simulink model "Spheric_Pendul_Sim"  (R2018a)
settings: Solver=ode8  StartTime=0.0  StopTime=80  FixedStep=Ts  MaxStep=0.0001  RelTol=1e-6  EnableMultiTasking=on
InitFcn:
  | init
StopFcn:
  | pl2
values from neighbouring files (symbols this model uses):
  Ax = 54.8    [init.m]
  d2r = pi/180    (= 0.0174532925199)    [init.m]
  Ixx = 3561    [init.m]
  Iyy = 20921    [init.m]
  Izz = 20763    [init.m]
  Mlh2 = 41.12    [init.m]
  Mlox = 119.3    [init.m]
  phi0 = 45*d2r    (= 0.785398163397)    [init.m]
  phid0 = 200.0*d2r    (= 3.49065850399)    [init.m]
  Rsl = 2.5    [init.m]
  thet0 = 18.0*d2r    (= 0.314159265359)    [init.m]
  Thr = 3.0    (= 3)    [init.m]
  x1_ini = [-1,0, -2,0, 2,0]*d2r    [init.m]
  x3_ini = [x1_ini,x3_ini]    [init.m]
  Xcg = 91.75    [init.m]
  Ys0 = R0*cos(phi0)    [init.m]
  Zeta = 0.002    [init.m]
  Zs0 = -R0*sin(phi0)    [init.m]
undefined symbols (not defined in the file or in its folder): Av2, Bv2, Cv2, Dv2, Kmix, Kq

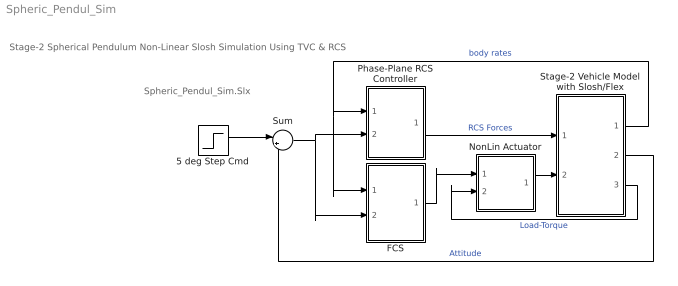
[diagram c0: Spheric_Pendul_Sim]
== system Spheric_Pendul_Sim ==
  note: Stage-2 Spherical Pendulum Non-Linear Slosh Simulation Using TVC & RCS
  note: Spheric_Pendul_Sim.Slx
  5 deg Step Cmd : Step  Time=0  Before=[0,0,0]  After=[1, 1, -1]*d2r*5  SampleTime=0
  FCS : Subsystem
  NonLin Actuator : Subsystem
  Phase-Plane RCS Controller : Subsystem
  Stage-2 Vehicle Model with Slosh/Flex : Subsystem
  Sum : Sum  Inputs=|+-
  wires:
  Stage-2 Vehicle Model with Slosh/Flex/1(Wb) -> Phase-Plane RCS Controller/1(rate), FCS/1(rate)  "body rates"
  Sum/1 -> Phase-Plane RCS Controller/2(atter), FCS/2(atter)
  Stage-2 Vehicle Model with Slosh/Flex/2(atti) -> Sum/2  "Attitude"
  FCS/1(DQ,DR) -> NonLin Actuator/1(dc)
  5 deg Step Cmd/1 -> Sum/1
  Stage-2 Vehicle Model with Slosh/Flex/3(TL) -> NonLin Actuator/2(TL)  "Load-Torque"
  Phase-Plane RCS Controller/1(f(i)) -> Stage-2 Vehicle Model with Slosh/Flex/1(Frcs)  "RCS Forces"
  NonLin Actuator/1(del) -> Stage-2 Vehicle Model with Slosh/Flex/2(dy,dz)

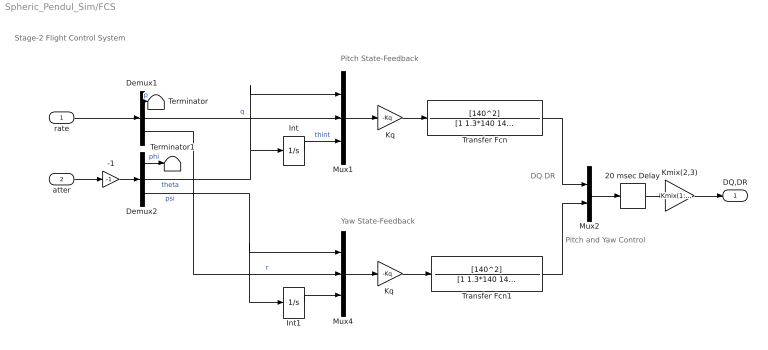
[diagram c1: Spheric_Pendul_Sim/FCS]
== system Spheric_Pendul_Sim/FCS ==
  note: DQ DR
  note: Pitch State-Feedback
  note: Yaw State-Feedback
  note: Pitch and Yaw Control
  note: Stage-2 Flight Control System
  rate : Inport
  atter : Inport  Port=2
  -1 : Gain  Gain=-1
  20 msec Delay : TransportDelay  DelayTime="[1  1]*0.020"  InitialOutput=[0 0]  PadeOrder=2
  Demux1 : Demux  Outputs=3
  Demux2 : Demux  Outputs=3
  Int : Integrator
  Int1 : Integrator
  Kmix(2,3) : Gain  Gain=Kmix(1:2,2:3)  Multiplication=Matrix(K*u)
  Kq : Gain  Gain=-Kq  Multiplication=Matrix(K*u)
  "Kq " : Gain  Gain=-Kq  Multiplication=Matrix(K*u)
  Mux1 : Mux  Inputs=3
  Mux2 : Mux  Inputs=2
  Mux4 : Mux  Inputs=3
  Terminator : Terminator
  Terminator1 : Terminator
  Transfer Fcn : TransferFcn  Numerator=[140^2]  Denominator=[1 1.3*140 140^2]
  Transfer Fcn1 : TransferFcn  Numerator=[140^2]  Denominator=[1 1.3*140 140^2]
  DQ,DR : Outport
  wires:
  Mux2/1 -> 20 msec Delay/1
  rate/1 -> Demux1/1
  Kq/1 -> Transfer Fcn/1
  Demux2/2 -> Mux1/1, Int/1  "theta"
  Demux1/2 -> Mux1/2  "q"
  Int/1 -> Mux1/3  "thint"
  Int1/1 -> Mux4/3
  Demux1/3 -> Mux4/2  "r"
  Demux2/3 -> Int1/1, Mux4/1  "psi"
  atter/1 -> -1/1
  Mux1/1 -> Kq/1
  Transfer Fcn/1 -> Mux2/1
  Transfer Fcn1/1 -> Mux2/2
  Mux4/1 -> "Kq "/1
  "Kq "/1 -> Transfer Fcn1/1
  Demux1/1 -> Terminator/1  "p"
  Demux2/1 -> Terminator1/1  "phi"
  20 msec Delay/1 -> Kmix(2,3)/1
  -1/1 -> Demux2/1
  Kmix(2,3)/1 -> DQ,DR/1

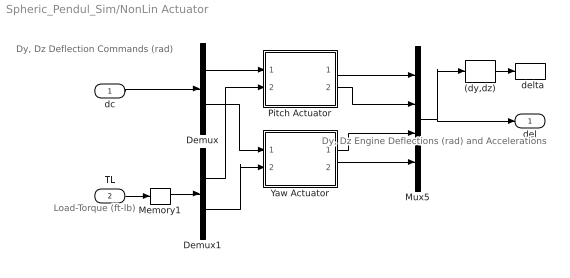
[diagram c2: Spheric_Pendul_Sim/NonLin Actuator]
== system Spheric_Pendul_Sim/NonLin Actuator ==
  note: Load-Torque (ft-lb)
  note: Dy, Dz Deflection Commands (rad)
  note: Dy, Dz Engine Deflections (rad) and Accelerations
  dc : Inport
  TL : Inport  Port=2
  "  delta" : ToWorkspace  VariableName=delta  SampleTime=-1
  (dy,dz) : Selector  InputPortWidth=4  IndexOptions=Index vector (dialog)  Indices=[1,3]  OutputSizes=1
  Demux : Demux  Outputs=2
  Demux1 : Demux  Outputs=2
  Memory1 : Memory
  Mux5 : Mux
  Pitch Actuator : Subsystem
  Yaw Actuator : Subsystem
  del : Outport
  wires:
  TL/1 -> Memory1/1
  dc/1 -> Demux/1
  Yaw Actuator/2(ddot) -> Mux5/4
  Demux/1 -> Pitch Actuator/1(delc)
  Pitch Actuator/2(ddot) -> Mux5/2
  Demux/2 -> Yaw Actuator/1(delc)
  Demux1/2 -> Yaw Actuator/2(TL)
  Mux5/1 -> del/1, (dy,dz)/1
  Demux1/1 -> Pitch Actuator/2(TL)
  (dy,dz)/1 -> "  delta"/1
  Memory1/1 -> Demux1/1
  Yaw Actuator/1(del) -> Mux5/3
  Pitch Actuator/1(del) -> Mux5/1

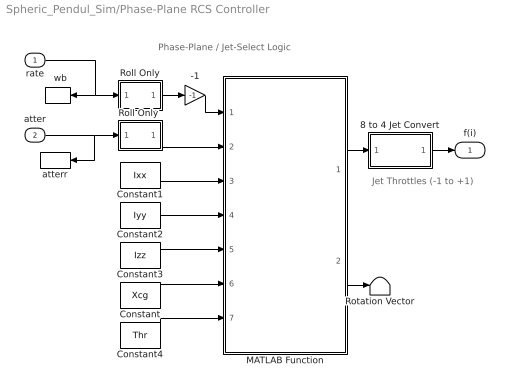
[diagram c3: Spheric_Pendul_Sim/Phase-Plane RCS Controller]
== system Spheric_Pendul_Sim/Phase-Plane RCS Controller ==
  note: Phase-Plane / Jet-Select Logic
  note: Jet Throttles (-1 to +1)
  rate : Inport
  atter : Inport  Port=2
  "  wb" : ToWorkspace  VariableName=wb  SampleTime=-1
  -1 : Gain  Gain=-1
  8 to 4 Jet Convert : Subsystem
  Constant : Constant  Value=Xcg
  Constant1 : Constant  Value=Ixx
  Constant2 : Constant  Value=Iyy
  Constant3 : Constant  Value=Izz
  Constant4 : Constant  Value=Thr
  MATLAB Function : MATLAB Function  TreatAsAtomicUnit=on
  Roll Only : Subsystem
  "Roll Only " : Subsystem
  Rotation Vector : Terminator
  atterr : ToWorkspace  VariableName=atter  SampleTime=-1
  f(i) : Outport
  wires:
  MATLAB Function/2(eu) -> Rotation Vector/1
  Constant4/1 -> MATLAB Function/7(Thr)
  Constant3/1 -> MATLAB Function/5(J33)
  8 to 4 Jet Convert/1(f(4)) -> f(i)/1
  MATLAB Function/1(fp) -> 8 to 4 Jet Convert/1(f(8))
  Constant2/1 -> MATLAB Function/4(J22)
  Constant1/1 -> MATLAB Function/3(J11)
  rate/1 -> "  wb"/1, Roll Only/1(w)
  Constant/1 -> MATLAB Function/6(Xcg)
  -1/1 -> MATLAB Function/1(Rater)
  Roll Only/1(p) -> -1/1
  "Roll Only "/1(p) -> MATLAB Function/2(Atter)
  atter/1 -> "Roll Only "/1(w), atterr/1

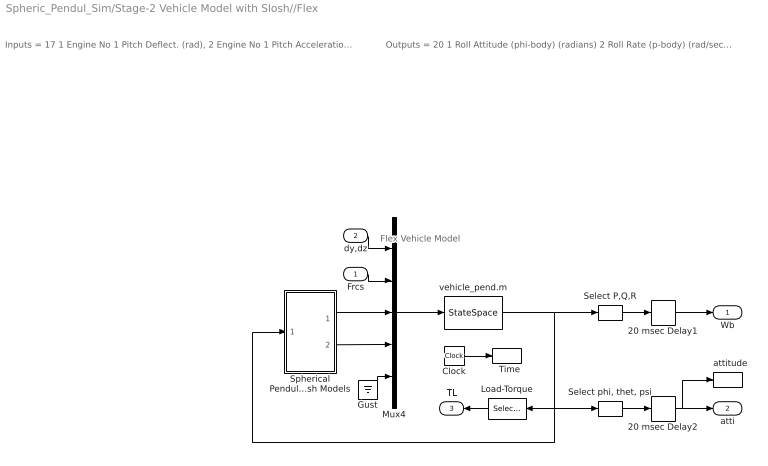
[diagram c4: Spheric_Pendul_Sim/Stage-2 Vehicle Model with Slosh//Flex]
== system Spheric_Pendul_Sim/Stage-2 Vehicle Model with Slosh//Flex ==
  note: Flex Vehicle Model
  note: Inputs = 17 1 Engine No 1 Pitch Deflect. (rad), 2 Engine No 1 Pitch Acceleration (rad/sec^2) 3 Engine No 1 Yaw Deflect. (rad), 4 Engine No 1 Yaw Acceleration (rad/sec^2) 5 RCS 1 Throttle Input dTh/Th 6 RCS 2 Throttle Input dTh/Th 7 RCS 3 Throttle Input dTh/Th 8 RCS 4 Throttle Input dTh/Th 9 LOX Force along Y-axis 10 LOX Force along Z-axis 11 LH2 Force along Y-axis 12 LH2 Force along Z-axis 13 Ext LOX Pitch Torque Inp 1 (ft-lb) 14 Ext LOX Yaw Torque Input 2 (ft-lb) 15 Ext LH2 Pitch Torque Inp 3 (ft-lb) 16 Ext LH2 Yaw Torque Input 4 (ft-lb) 17 Wind Gust Velocity (ft/sec)
  note: Outputs = 20 1 Roll Attitude (phi-body) (radians) 2 Roll Rate (p-body) (rad/sec) 3 Pitch Attitude (thet-bdy) (radians) 4 Pitch Rate (q-body) (rad/sec) 5 Yaw Attitude (psi-body) (radians) 6 Yaw Rate (r-body) (rad/sec) 7 Angle of attack, alfa, (radians) 8 Angle of sideslip, beta, (radian) 9 Change in Altitude, delta-h, (feet) 10 Forward Acceleration (V-dot) (ft/sec) 11 Cross Range Velocity (Vcr) (ft/sec) 12 Rate-Gyro # 1, Roll Rate (Body) (rad/sec) 13 Rate-Gyro # 2, Pitch Rate (Body) (rad/sec) 14 Rate-Gyro # 3, Yaw Rate (Body) (rad/sec) 15 Accelerat # 1, at LOX (along Y), (ft/sec^2) 16 Accelerat # 2, at LOX (along Z), (ft/sec^2) 17 Accelerat # 3, at LH2 (along Y), (ft/sec^2) 18 Accelerat # 4, at LH2 (along Z), (ft/sec^2) 19 Ptch Engine Load-Torque Tly (ft-lb) 20 Yaw Engine Load-Torque Tlz (ft-lb)
  Frcs : Inport
  dy,dz : Inport  Port=2
  "  Time" : ToWorkspace  VariableName=tim  SampleTime=-1
  "  attitude" : ToWorkspace  VariableName=atti  SampleTime=-1
  20 msec Delay1 : TransportDelay  DelayTime=[1 1 1]*0.02  InitialOutput=[0 0 0]  PadeOrder=2
  20 msec Delay2 : TransportDelay  DelayTime=[1 1 1]*0.02  InitialOutput=x1_ini([1,3,5])  PadeOrder=2
  Clock : Clock
  Gust : Ground
  Load-Torque : Selector  InputPortWidth=20  IndexOptions=Index vector (dialog)  Indices=[19, 20]  OutputSizes=1
  Mux4 : Mux  Inputs=[4,4,4,4,1]
  Select P,Q,R : Selector  InputPortWidth=20  IndexOptions=Index vector (dialog)  Indices=[12,13,14]  OutputSizes=1
  "Select phi, thet, psi" : Selector  InputPortWidth=20  IndexOptions=Index vector (dialog)  Indices=[1,3,5]  OutputSizes=1
  Spherical Pendulum Slosh Models : Subsystem
  vehicle_pend.m : StateSpace  A=Av2  B=Bv2  C=Cv2  D=Dv2  InitialCondition=x3_ini
  Wb : Outport
  atti : Outport  Port=2
  TL : Outport  Port=3
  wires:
  Gust/1 -> Mux4/5
  Frcs/1 -> Mux4/2
  dy,dz/1 -> Mux4/1
  Load-Torque/1 -> TL/1
  Clock/1 -> "  Time"/1
  20 msec Delay2/1 -> "  attitude"/1, atti/1
  20 msec Delay1/1 -> Wb/1
  vehicle_pend.m/1 -> Select P,Q,R/1, "Select phi, thet, psi"/1, Spherical Pendulum Slosh Models/1(Ayz), Load-Torque/1
  Spherical Pendulum Slosh Models/1(Fyz) -> Mux4/3
  Spherical Pendulum Slosh Models/2(Myz) -> Mux4/4
  Select P,Q,R/1 -> 20 msec Delay1/1
  "Select phi, thet, psi"/1 -> 20 msec Delay2/1
  Mux4/1 -> vehicle_pend.m/1

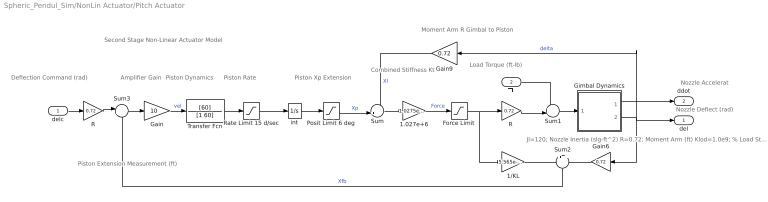
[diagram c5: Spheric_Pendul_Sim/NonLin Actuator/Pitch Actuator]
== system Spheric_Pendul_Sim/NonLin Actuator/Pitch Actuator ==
  note: Jl=120; Nozzle Inertia (slg-ft^2) R=0.72; Moment Arm (ft) Klod=1.0e9; % Load Stiffness Kact=2.4e6; % Piston Stiffness Kbck=1.13e6; % Backup Structure Stiffn Kti=(1/Klod)+(1/Kact)+(1/Kbck); Kt=1/Kti; % Combined Structural Stiffness Ka=8; % Amplifier Gain
  note: Load Torque (ft-lb)
  note: Deflection Command (rad)
  note: Piston Xp Extension
  note: Combined Stiffness Kt
  note: Piston Dynamics
  note: Nozzle Accelerat
  note: Nozzle Deflect (rad)
  note: Amplifier Gain
  note: Piston Rate
  note: Second Stage Non-Linear Actuator Model
  note: Moment Arm R Gimbal to Piston
  note: Piston Extension Measurement (ft)
  delc : Inport
  TL : Inport  Port=2
  1.027e+6 : Gain  Gain=1.0275e+6
  1/KL : Gain  Gain=5.565e-07
  Force Limit : Saturate  UpperLimit=4000  LowerLimit=-4000
  Gain : Gain  Gain=10
  Gain6 : Gain  Gain=0.72
  Gain9 : Gain  Gain=0.72
  Gimbal Dynamics : Subsystem
  Posit Limit 6 deg : Saturate  UpperLimit=0.075  LowerLimit=-0.075
  R : Gain  Gain=0.72
  "R " : Gain  Gain=0.72
  Rate Limit 15 d/sec : Saturate  UpperLimit=0.125  LowerLimit=-0.125
  Sum : Sum  Inputs=-+|
  Sum1 : Sum  Inputs=++|
  Sum2 : Sum  Inputs=+|+
  Sum3 : Sum  Inputs=|+-
  Transfer Fcn : TransferFcn  Numerator=[60]  Denominator=[1 60]
  int : Integrator
  del : Outport
  ddot : Outport  Port=2
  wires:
  Transfer Fcn/1 -> Rate Limit 15 d/sec/1
  Sum1/1 -> Gimbal Dynamics/1(Tin)
  Gimbal Dynamics/1(Axel) -> ddot/1
  Posit Limit 6 deg/1 -> Sum/2  "Xp"
  1/KL/1 -> Sum2/1
  Gain9/1 -> Sum/1  "Xl"
  1.027e+6/1 -> Force Limit/1  "Force"
  Gain6/1 -> Sum2/2
  Rate Limit 15 d/sec/1 -> int/1
  Gain/1 -> Transfer Fcn/1  "vel"
  Sum3/1 -> Gain/1
  Sum/1 -> 1.027e+6/1
  int/1 -> Posit Limit 6 deg/1
  TL/1 -> Sum1/1
  R/1 -> Sum3/1
  delc/1 -> R/1
  Force Limit/1 -> "R "/1, 1/KL/1
  "R "/1 -> Sum1/2
  Gimbal Dynamics/2(" delta") -> Gain9/1, del/1, Gain6/1  "delta"
  Sum2/1 -> Sum3/2  "Xfb"

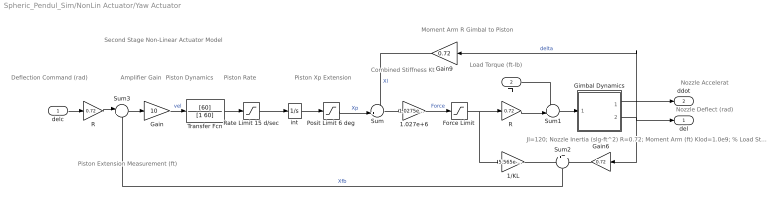
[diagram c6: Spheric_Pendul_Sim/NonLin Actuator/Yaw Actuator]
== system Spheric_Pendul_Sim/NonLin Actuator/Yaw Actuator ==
  note: Jl=120; Nozzle Inertia (slg-ft^2) R=0.72; Moment Arm (ft) Klod=1.0e9; % Load Stiffness Kact=2.4e6; % Piston Stiffness Kbck=1.13e6; % Backup Structure Stiffn Kti=(1/Klod)+(1/Kact)+(1/Kbck); Kt=1/Kti; % Combined Structural Stiffness Ka=8; % Amplifier Gain
  note: Load Torque (ft-lb)
  note: Deflection Command (rad)
  note: Piston Xp Extension
  note: Combined Stiffness Kt
  note: Piston Dynamics
  note: Nozzle Accelerat
  note: Nozzle Deflect (rad)
  note: Amplifier Gain
  note: Piston Rate
  note: Second Stage Non-Linear Actuator Model
  note: Moment Arm R Gimbal to Piston
  note: Piston Extension Measurement (ft)
  delc : Inport
  TL : Inport  Port=2
  1.027e+6 : Gain  Gain=1.0275e+6
  1/KL : Gain  Gain=5.565e-07
  Force Limit : Saturate  UpperLimit=4000  LowerLimit=-4000
  Gain : Gain  Gain=10
  Gain6 : Gain  Gain=0.72
  Gain9 : Gain  Gain=0.72
  Gimbal Dynamics : Subsystem
  Posit Limit 6 deg : Saturate  UpperLimit=0.075  LowerLimit=-0.075
  R : Gain  Gain=0.72
  "R " : Gain  Gain=0.72
  Rate Limit 15 d/sec : Saturate  UpperLimit=0.125  LowerLimit=-0.125
  Sum : Sum  Inputs=-+|
  Sum1 : Sum  Inputs=++|
  Sum2 : Sum  Inputs=+|+
  Sum3 : Sum  Inputs=|+-
  Transfer Fcn : TransferFcn  Numerator=[60]  Denominator=[1 60]
  int : Integrator
  del : Outport
  ddot : Outport  Port=2
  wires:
  Transfer Fcn/1 -> Rate Limit 15 d/sec/1
  Sum1/1 -> Gimbal Dynamics/1(Tin)
  Gimbal Dynamics/1(Axel) -> ddot/1
  Posit Limit 6 deg/1 -> Sum/2  "Xp"
  1/KL/1 -> Sum2/1
  Gain9/1 -> Sum/1  "Xl"
  1.027e+6/1 -> Force Limit/1  "Force"
  Gain6/1 -> Sum2/2
  Rate Limit 15 d/sec/1 -> int/1
  Gain/1 -> Transfer Fcn/1  "vel"
  Sum3/1 -> Gain/1
  Sum/1 -> 1.027e+6/1
  int/1 -> Posit Limit 6 deg/1
  TL/1 -> Sum1/1
  R/1 -> Sum3/1
  delc/1 -> R/1
  Force Limit/1 -> "R "/1, 1/KL/1
  "R "/1 -> Sum1/2
  Gimbal Dynamics/2(" delta") -> Gain9/1, del/1, Gain6/1  "delta"
  Sum2/1 -> Sum3/2  "Xfb"

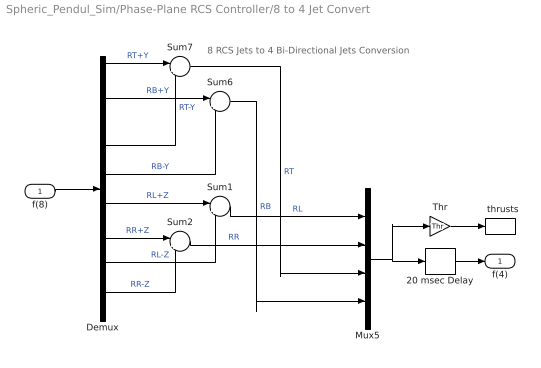
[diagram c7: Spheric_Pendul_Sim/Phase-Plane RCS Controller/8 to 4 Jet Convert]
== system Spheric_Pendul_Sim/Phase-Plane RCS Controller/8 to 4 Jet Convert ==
  note: 8 RCS Jets to 4 Bi-Directional Jets Conversion
  f(8) : Inport
  "  thrusts" : ToWorkspace  VariableName=Jets  SampleTime=-1
  20 msec Delay : TransportDelay  DelayTime="[1  1  1  1]*0.020"  InitialOutput="[0  0  0  0]"  PadeOrder=2
  Demux : Demux  Outputs=8
  Mux5 : Mux
  Sum{1..2,6..7} (4 alike) : Sum  Inputs=|+-
  Thr : Gain  Gain=Thr
  f(4) : Outport
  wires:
  Thr/1 -> "  thrusts"/1
  20 msec Delay/1 -> f(4)/1
  Sum2/1 -> Mux5/2  "RR"
  Sum1/1 -> Mux5/1  "RL"
  Demux/4 -> Sum6/2  "RB-Y"
  Demux/2 -> Sum6/1  "RB+Y"
  Demux/3 -> Sum7/2  "RT-Y"
  Sum7/1 -> Mux5/3  "RT"
  Demux/8 -> Sum2/2  "RR-Z"
  Demux/5 -> Sum1/1  "RL+Z"
  Sum6/1 -> Mux5/4  "RB"
  Demux/1 -> Sum7/1  "RT+Y"
  Demux/6 -> Sum2/1  "RR+Z"
  Demux/7 -> Sum1/2  "RL-Z"
  Mux5/1 -> Thr/1, 20 msec Delay/1
  f(8)/1 -> Demux/1

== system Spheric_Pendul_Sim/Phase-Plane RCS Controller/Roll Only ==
  w : Inport
  Ground : Ground
  Mux : Mux  Inputs=3
  Selector : Selector  InputPortWidth=3  IndexOptions=Index vector (dialog)  Indices=[1]  OutputSizes=1
  p : Outport
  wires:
  Ground/1 -> Mux/2, Mux/3
  Selector/1 -> Mux/1
  Mux/1 -> p/1
  w/1 -> Selector/1

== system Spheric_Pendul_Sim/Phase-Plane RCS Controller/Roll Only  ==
  w : Inport
  Ground : Ground
  Mux : Mux  Inputs=3
  Selector : Selector  InputPortWidth=3  IndexOptions=Index vector (dialog)  Indices=[1]  OutputSizes=1
  p : Outport
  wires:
  Ground/1 -> Mux/2, Mux/3
  Selector/1 -> Mux/1
  Mux/1 -> p/1
  w/1 -> Selector/1

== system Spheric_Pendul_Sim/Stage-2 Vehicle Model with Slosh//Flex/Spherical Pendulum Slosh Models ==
  note: Spherical Pendulum Slosh Modes
  Ayz : Inport
  LH2 Slosh : Subsystem
  LOX Slosh : Subsystem
  Mux1 : Mux  Inputs=[2, 2]
  Mux2 : Mux  Inputs=[2, 2]
  Fyz : Outport
  Myz : Outport  Port=2
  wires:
  Mux1/1 -> Fyz/1
  LOX Slosh/1(Fox) -> Mux1/1
  LH2 Slosh/1(Fh2) -> Mux1/2
  LOX Slosh/2(Mox) -> Mux2/1
  LH2 Slosh/2(Mh2) -> Mux2/2
  Mux2/1 -> Myz/1
  Ayz/1 -> LH2 Slosh/1(Ayz), LOX Slosh/1(Ayz)

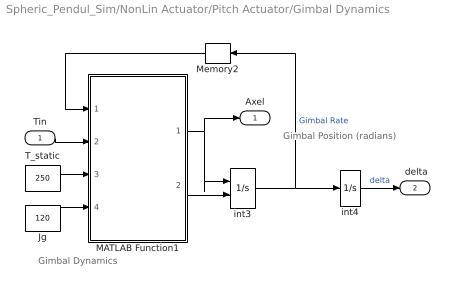
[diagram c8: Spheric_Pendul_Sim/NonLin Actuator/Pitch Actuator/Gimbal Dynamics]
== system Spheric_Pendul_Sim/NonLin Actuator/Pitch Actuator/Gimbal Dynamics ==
  note: Gimbal Dynamics
  note: Gimbal Position (radians)
  Tin : Inport
  Jg : Constant  Value=120
  MATLAB Function1 : MATLAB Function  TreatAsAtomicUnit=on
  Memory2 : Memory
  T_static : Constant  Value=250
  int3 : Integrator  ExternalReset=rising
  int4 : Integrator
  Axel : Outport
  " delta" : Outport  Port=2
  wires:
  Memory2/1 -> MATLAB Function1/1(Rate)
  Jg/1 -> MATLAB Function1/4(Jg)
  MATLAB Function1/1(Axel) -> int3/1, Axel/1
  T_static/1 -> MATLAB Function1/3(Tst)
  Tin/1 -> MATLAB Function1/2(Tin)
  int3/1 -> Memory2/1, int4/1  "Gimbal Rate"
  int4/1 -> " delta"/1  "delta"
  MATLAB Function1/2(Rvel) -> int3/2

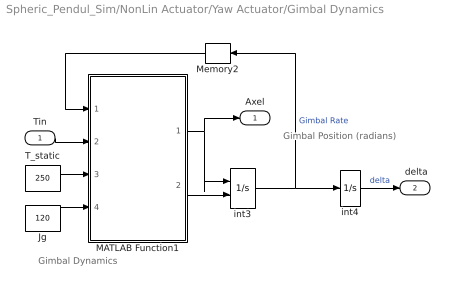
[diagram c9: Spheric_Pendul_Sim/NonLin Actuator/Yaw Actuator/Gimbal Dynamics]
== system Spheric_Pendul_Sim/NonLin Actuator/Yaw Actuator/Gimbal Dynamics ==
  note: Gimbal Dynamics
  note: Gimbal Position (radians)
  Tin : Inport
  Jg : Constant  Value=120
  MATLAB Function1 : MATLAB Function  TreatAsAtomicUnit=on
  Memory2 : Memory
  T_static : Constant  Value=250
  int3 : Integrator  ExternalReset=rising
  int4 : Integrator
  Axel : Outport
  " delta" : Outport  Port=2
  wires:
  Memory2/1 -> MATLAB Function1/1(Rate)
  Jg/1 -> MATLAB Function1/4(Jg)
  MATLAB Function1/1(Axel) -> int3/1, Axel/1
  T_static/1 -> MATLAB Function1/3(Tst)
  Tin/1 -> MATLAB Function1/2(Tin)
  int3/1 -> Memory2/1, int4/1  "Gimbal Rate"
  int4/1 -> " delta"/1  "delta"
  MATLAB Function1/2(Rvel) -> int3/2

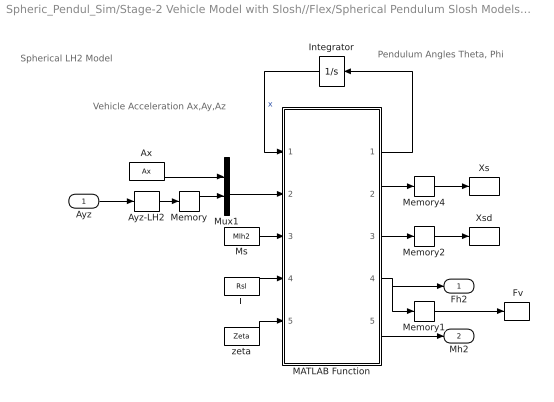
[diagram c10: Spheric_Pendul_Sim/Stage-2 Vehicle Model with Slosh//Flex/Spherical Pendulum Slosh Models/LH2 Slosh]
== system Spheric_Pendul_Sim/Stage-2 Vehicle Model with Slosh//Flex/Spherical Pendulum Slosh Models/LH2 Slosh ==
  note: Spherical LH2 Model
  note: Vehicle Acceleration Ax,Ay,Az
  note: Pendulum Angles Theta, Phi
  Ayz : Inport
  " Fv" : ToWorkspace  VariableName=Fvb  SampleTime=-1
  " Xs " : ToWorkspace  VariableName=Xsb  SampleTime=-1
  " Xsd " : ToWorkspace  VariableName=Xsdb  SampleTime=-1
  Ax : Constant  Value=Ax
  Ayz-LH2 : Selector  InputPortWidth=20  IndexOptions=Index vector (dialog)  Indices=[17,18]  OutputSizes=1
  Integrator : Integrator  InitialCondition=[0,phid0, thet0,phi0]
  L : Constant  Value=Rsl
  MATLAB Function : MATLAB Function  TreatAsAtomicUnit=on
  Memory : Memory
  Memory1 : Memory
  Memory2 : Memory
  Memory4 : Memory  InitialCondition=[Ys0,Zs0]
  Ms : Constant  Value=Mlh2
  Mux1 : Mux  Inputs=[1, 2]
  zeta : Constant  Value=Zeta
  Fh2 : Outport
  Mh2 : Outport  Port=2
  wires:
  MATLAB Function/5(Mv) -> Mh2/1
  MATLAB Function/4(Fv) -> Fh2/1, Memory1/1
  L/1 -> MATLAB Function/4(Rsl)
  zeta/1 -> MATLAB Function/5(zeta)
  Ms/1 -> MATLAB Function/3(Msl)
  Mux1/1 -> MATLAB Function/2(Acc)
  MATLAB Function/1(xdot) -> Integrator/1
  Integrator/1 -> MATLAB Function/1(x)  "x"
  MATLAB Function/2(Xs) -> Memory4/1
  MATLAB Function/3(Xsd) -> Memory2/1
  Memory1/1 -> " Fv"/1
  Memory4/1 -> " Xs "/1
  Memory2/1 -> " Xsd "/1
  Ayz/1 -> Ayz-LH2/1
  Ax/1 -> Mux1/1
  Ayz-LH2/1 -> Memory/1
  Memory/1 -> Mux1/2

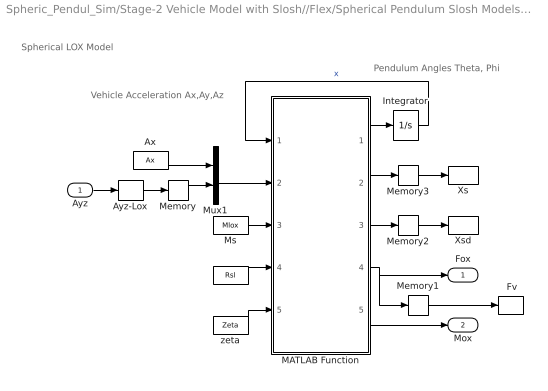
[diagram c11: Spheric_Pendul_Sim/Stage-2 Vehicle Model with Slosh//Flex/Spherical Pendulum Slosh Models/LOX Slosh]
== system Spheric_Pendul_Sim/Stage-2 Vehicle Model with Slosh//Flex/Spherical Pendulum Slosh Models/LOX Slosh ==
  note: Spherical LOX Model
  note: Vehicle Acceleration Ax,Ay,Az
  note: Pendulum Angles Theta, Phi
  Ayz : Inport
  " Fv" : ToWorkspace  VariableName=Fva  SampleTime=-1
  " Xs " : ToWorkspace  VariableName=Xsa  SampleTime=-1
  " Xsd " : ToWorkspace  VariableName=Xsda  SampleTime=-1
  Ax : Constant  Value=Ax
  Ayz-Lox : Selector  InputPortWidth=20  IndexOptions=Index vector (dialog)  Indices=[15,16]  OutputSizes=1
  Integrator : Integrator  InitialCondition=[0,phid0, thet0,phi0]
  L : Constant  Value=Rsl
  MATLAB Function : MATLAB Function  TreatAsAtomicUnit=on
  Memory : Memory
  Memory1 : Memory
  Memory2 : Memory
  Memory3 : Memory  InitialCondition=[Ys0, Zs0]
  Ms : Constant  Value=Mlox
  Mux1 : Mux  Inputs=[1, 2]
  zeta : Constant  Value=Zeta
  Fox : Outport
  Mox : Outport  Port=2
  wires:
  MATLAB Function/5(Mv) -> Mox/1
  MATLAB Function/4(Fv) -> Fox/1, Memory1/1
  L/1 -> MATLAB Function/4(Rsl)
  zeta/1 -> MATLAB Function/5(zeta)
  Ms/1 -> MATLAB Function/3(Msl)
  Mux1/1 -> MATLAB Function/2(Acc)
  MATLAB Function/1(xdot) -> Integrator/1
  Integrator/1 -> MATLAB Function/1(x)  "x"
  MATLAB Function/2(Xs) -> Memory3/1
  MATLAB Function/3(Xsd) -> Memory2/1
  Memory1/1 -> " Fv"/1
  Memory3/1 -> " Xs "/1
  Memory2/1 -> " Xsd "/1
  Ax/1 -> Mux1/1
  Ayz/1 -> Ayz-Lox/1
  Ayz-Lox/1 -> Memory/1
  Memory/1 -> Mux1/2

== matlab function Spheric_Pendul_Sim/Stage-2
Vehicle Model 
with Slosh//Flex/Spherical
Pendulum
Slosh Models/LOX Slosh/MATLAB Function ==
function [xdot,Xs,Xsd,Fv,Mv]= Spherical_Pend(x,Acc,Msl,Rsl,zeta) 
% Spherical Pendulum Slosh Model  
% [xdot,Xs,Xsd,Fv,Mv]= Spherical_Pend(x,Acc,Msl,Rsl,zeta)   
% Calculates the Slosh Forces on the Tank as a function of 
% Vehicle acceleration at the Tank
%
% State Variables (x) 
% x(1:2)  = Xsd Slosh Mass Ysd,Zsd Velocity wrt Tank 
% x(3:4)  = Xs Slosh Mass Ys,Zs Position wrt Tank 
% Acc(3}  = Vehicle Linear Ax,Ay,Az Accelerat at Tank
% Msl     = Slosh Mass (slug)
% Rsl     = Pendulum length (ft)
 
xdot=zeros(4,1);                                      % Initialize
thd= x(1);                                            % Theta-dot
phd= x(2);                                            % Phi-dot
the= x(3);                                            % Theta
phi= x(4);                                            % Phi
Ax= Acc(1);                                           % Y-accelerat at Tank
Ay= Acc(2);                                           % Y-accelerat at Tank
Az= Acc(3);                                           % Z-accelerat at Tank
Wsl=sqrt(Ax/Rsl);                                     % Slosh Frequency (r/s)
Sth=sin(the); Cth=cos(the); 
Sph=sin(phi); Cph=cos(phi); 
if abs(Sth)< 1.e-7                                    % Avoid Singularity
    Sth=1.e-7*sign(Sth);
end

% Axial and Tangential Accelerations
Aksi= Ay*Cph - Az*Sph;                                % Axial   Accel
Atau= Az*Cph + Ay*Sph;                                % Tangent Accel

% Vertical and Horizontal Accelerations
thdd=(phd^2)*Cth*Sth -(Ax/Rsl)*Sth -(Aksi/Rsl)*Cth -2*zeta*Wsl*thd;
phdd=-2*thd*phd*(Cth/Sth) + Atau/(Rsl*Sth) -2*zeta*Wsl*phd;
 
% Slosh Mass Displacements Relative to Tank Ys, Zs
%Xs=-Rsl*Cth;
Ys= Rsl*Sth*Cph;
Zs=-Rsl*Sth*Sph; Xs=[Ys;Zs];

% Slosh Mass Velocities Relative to Tank Ys, Zs
Ysd= Rsl*(thd*Cth*Cph - phd*Sth*Sph);
Zsd=-Rsl*(thd*Cth*Sph + phd*Sth*Cph); Xsd=[Ysd;Zsd];

% Slosh Mass Accelerations Relative to Tank Ysd, Zsd
Ysdd= Rsl*(+thdd*Cth*Cph - phdd*Sth*Sph -2*thd*phd*Cth*Sph -(thd^2+phd^2)*Sth*Cph);
Zsdd= Rsl*(-thdd*Cth*Sph - phdd*Sth*Cph -2*thd*phd*Cth*Cph +(thd^2+phd^2)*Sth*Sph);
 
% Lateral Forces on the Vehicle = Mass x Inert Acceleration
Fv=-Msl*([Ysdd+Ay; Zsdd+Az]);                         % Forces on the Vehicle
Mv= Msl*Ax*[-Zs; Ys];                                 % Additional Moments due to Ax
 
% State Derivatives 
xdot(1:2)= [thdd;phdd];                               % X-dot-dot 
xdot(3:4)= [thd; phd];                                % X-dot[4]
end

== matlab function Spheric_Pendul_Sim/Phase-Plane
RCS Controller/MATLAB Function ==
function [fp, eu]= Phase_Plane(Rater,Atter, J11,J22,J33, Xcg,Thr)    
% Phase-Plane Logic for RCS jets
% Rater: Rate Error in (deg/sec)
% Atter: Attitude Error in (deg)

% Define Phase-Plane Logic Parameters in (deg)
r2d=180/pi;
nt=8;                                                    % Number of Jets
cg2= [Xcg, 0.0, 0.0]';                                   % CG Location
ang_acl     = Thr*150*[6/J11, 20/J22, 20/J33];
att_deadband= [1, 1, 1]*0.5; 
kledge      = [1, 1, 1]*1.2; 
rate_lim    = [1, 1, 1]*6.0; 
low_rate_lim= rate_lim*0.31;

% RCS Thruster Directions ----------------------------------------------
Jdir= zeros(3,nt); Jloc=Jdir;
Jdir(:, 1)= [0.0,  +1.0,   0.0]';                         % Top   +Y
Jdir(:, 2)= [0.0,  +1.0,   0.0]';                         % Botm  +Y
Jdir(:, 3)= [0.0,  -1.0,   0.0]';                         % Top   -Y
Jdir(:, 4)= [0.0,  -1.0,   0.0]';                         % Botm  -Y
Jdir(:, 5)= [0.0,   0.0,  +1.0]';                         % Left  +Z
Jdir(:, 6)= [0.0,   0.0,  +1.0]';                         % Right +Z
Jdir(:, 7)= [0.0,   0.0,  -1.0]';                         % Left  -Z
Jdir(:, 8)= [0.0,   0.0,  -1.0]';                         % Right -Z

% RCS Thruster Locations -----------------------------------------------
Jloc(:, 1) = [83,  0.0, -3.5]';                           % Top   +Y
Jloc(:, 2) = [83,  0.0, +3.5]';                           % Botm  +Y
Jloc(:, 3) = [83,  0.0, -3.5]';                           % Top   -Y
Jloc(:, 4) = [83,  0.0, +3.5]';                           % Botm  -Y
Jloc(:, 5) = [83, -3.5,  0.0]';                           % Left  +Z
Jloc(:, 6) = [83, +3.5,  0.0]';                           % Right +Z
Jloc(:, 7) = [83, -3.5,  0.0]';                           % Left  -Z
Jloc(:, 8) = [83, +3.5,  0.0]';                           % Right -Z

rat_err= Rater*r2d;                                    % Convert to (deg)
att_err= Atter*r2d;
Cnt= [0;0;0];                                          % Control to JetSel

for iax=1:3
    sign_rat_err= sign(rat_err(iax)+1.0e-8);
    x1 = sign_rat_err*att_err(iax);
    x2 = abs(rat_err(iax));
    ang_acl_gain= 2*ang_acl(iax);
    curve = rat_err(iax)^2/ang_acl_gain;
    
    sw1= -curve + att_deadband(iax);
    sw2= -(curve + (kledge(iax)*att_deadband(iax)));
    sw3= rate_lim(iax);
    sw5= low_rate_lim(iax);
    
    if ((x1>sw1) || (x2>sw3)), Cnt(iax)= -sign_rat_err; % Region 1
    elseif (x1 >= sw2), Cnt(iax)= 0;                    % Region 2
    elseif (x2 < sw5), Cnt(iax)= sign_rat_err;          % Region 3
    else, Cnt(iax)= 0;  
    end
end

% Select Jets
if abs(Cnt)>0, eu= Cnt/sqrt(Cnt'*Cnt);                  % Direction Unit vect
else, eu=Cnt; end
fp= Jet_Select_dot(-eu,4, nt,Thr,cg2,Jloc,Jdir);        % Get Thruster Forces

function fp= Jet_Select_dot(eu,Imax, nt,Thr,cg2,Jloc,Jdir)
% fp= Jet_Select_dot(eu,nt,Thr,Jloc,Jdir,Imax)
% Compute the thrust force vector (fp)
% Inputs
% eu(3) : ACS error unit vector
% nt    : number of jets
% Thr   : Thrust in (lb)
% Jloc  : Jet Locations 
% Jdir  : Thrust directions
% Imax  : Max number of Thrusters to select
% J     : Vehicle MOI matrix (3x3)
% cg(3) : CG location
% Outputs
% fp(nt): Thrusts vector (nt)

if sqrt(eu'*eu)<0.9, fp=zeros(nt,1); return; end    % Direct must be unit vect

tm= Thr*ones(1,nt);
vt= zeros(3,nt); pf= zeros(nt,1); sf=pf;

% Select the most dominant jets from all of them
for i=1:nt
    ln= (Jloc(:,i) - cg2);                          % Moment arms
    vt(:,i)= tm(i)*cross(ln,Jdir(:,i));             % Moments Matrix using all jets
    pf(i) = dot(vt(:,i),eu);                        % Moment dotted with maneuv direct
end

f2=pf;
for i=1:(nt/2)
    [mf,sf(i)]=max(f2); f2(sf(i))=0;                % Identify the strongest half
end
pf= pf/pf(sf(1));                                   % Normlz relative to strongest

% Select Imax jets among the strongest
Isel=1;                                             % First, select the strongest
for i=1:Imax-1
    if pf(sf(i+1))>0.72; Isel=Isel+1; end            % 70% contrib, choose one more jet to Imax
end

fp= zeros(nt,1);                                    % Initially zero all jets
for i=1:nt
    for j=1:Isel
        if i==sf(j); fp(i)=1; end                   % Turn on the selected jet force
    end
end

== matlab function Spheric_Pendul_Sim/Stage-2
Vehicle Model 
with Slosh//Flex/Spherical
Pendulum
Slosh Models/LH2 Slosh/MATLAB Function ==
function [xdot,Xs,Xsd,Fv,Mv]= Spherical_Pend(x,Acc,Msl,Rsl,zeta) 
% Spherical Pendulum Slosh Model  
% [xdot,Xs,Xsd,Fv,Mv]= Spherical_Pend(x,Acc,Msl,Rsl,zeta)   
% Calculates the Slosh Forces on the Tank as a function of 
% Vehicle acceleration at the Tank
%
% State Variables (x) 
% x(1:2)  = Xsd Slosh Mass Ysd,Zsd Velocity wrt Tank 
% x(3:4)  = Xs Slosh Mass Ys,Zs Position wrt Tank 
% Acc(3}  = Vehicle Linear Ax,Ay,Az Accelerat at Tank
% Msl     = Slosh Mass (slug)
% Rsl     = Pendulum length (ft)
 
xdot=zeros(4,1);                                      % Initialize
thd= x(1);                                            % Theta-dot
phd= x(2);                                            % Phi-dot
the= x(3);                                            % Theta
phi= x(4);                                            % Phi
Ax= Acc(1);                                           % Y-accelerat at Tank
Ay= Acc(2);                                           % Y-accelerat at Tank
Az= Acc(3);                                           % Z-accelerat at Tank
Wsl=sqrt(Ax/Rsl);                                     % Slosh Frequency (r/s)
Sth=sin(the); Cth=cos(the); 
Sph=sin(phi); Cph=cos(phi); 
if abs(Sth)< 1.e-7 
    Sth=1.e-7*sign(Sth);
end

% Axial and Tangential Accelerations
Aksi= Ay*Cph - Az*Sph;                                % Axial   Accel
Atau= Az*Cph + Ay*Sph;                                % Tangent Accel

% Vertical and Horizontal Accelerations
thdd=(phd^2)*Cth*Sth -(Ax/Rsl)*Sth -(Aksi/Rsl)*Cth -2*zeta*Wsl*thd;
phdd=-2*thd*phd*(Cth/Sth) + Atau/(Rsl*Sth) -2*zeta*Wsl*phd;
 
% Slosh Mass Displacements Relative to Tank Ys, Zs
%Xs=-Rsl*Cth;
Ys= Rsl*Sth*Cph;
Zs=-Rsl*Sth*Sph; Xs=[Ys;Zs];

% Slosh Mass Velocities Relative to Tank Ys, Zs
Ysd= Rsl*(thd*Cth*Cph - phd*Sth*Sph);
Zsd=-Rsl*(thd*Cth*Sph + phd*Sth*Cph); Xsd=[Ysd;Zsd];

% Slosh Mass Accelerations Relative to Tank Ysd, Zsd
Ysdd= Rsl*(+thdd*Cth*Cph - phdd*Sth*Sph -2*thd*phd*Cth*Sph -(thd^2+phd^2)*Sth*Cph);
Zsdd= Rsl*(-thdd*Cth*Sph - phdd*Sth*Cph -2*thd*phd*Cth*Cph +(thd^2+phd^2)*Sth*Sph);
 
% Lateral Forces on the Vehicle = Mass x Inert Acceleration
Fv=-Msl*([Ysdd+Ay; Zsdd+Az]);                         % Forces on the Vehicle
Mv= Msl*Ax*[-Zs; Ys];                                 % Additional Moments due to Ax
 
% State Derivatives 
xdot(1:2)= [thdd;phdd];                               % X-dot-dot 
xdot(3:4)= [thd; phd];                                % X-dot[4]
end

== matlab function Spheric_Pendul_Sim/NonLin Actuator/Pitch Actuator/Gimbal 
Dynamics/MATLAB Function1 ==
function [Axel,Rvel] = Gimbal(Rate,Tin,Tst,Jg)    
% Gimbal Friction Dynamics
% Tin:  Input Torque (ft-lb)
% Rate: Gimbal Rate (rad/sec)
% Tfr:  Gimbal Friction Torque (ft-lb)
% axel: Gimbal Acceleration (ft/sec2)
% Tst:  Gimbal Static Friction Torq (ft-lb)
% Jg:   Gimbal Inertia (slg-ft^2)

if abs(Rate)<0.01                     % If Not Moving Much
    if abs(Tin)>Tst*1.05              % Exceeds Stiction, Start Moving
        Tfr=Tst*sign(Tin);            % Friction Torque resist motion
        Axel=(Tin-Tfr)/Jg;            % Gimbal Acceleration
        Rvel=0;
    else                              % Stop the Motion
        Axel=0;
        Tfr=0;                        % No Frict when not moving
        Rvel=1;                       % Reset Velocity to Zero
    end
    
else                                  % Gimbal is Fast Enough
    Tfr=Tst*sign(Rate);               % Friction Torque resist motion
    Axel=(Tin-Tfr)/Jg;                % Gimbal Acceleration
    Rvel=0;
end

== matlab function Spheric_Pendul_Sim/NonLin Actuator/Yaw Actuator/Gimbal 
Dynamics/MATLAB Function1 ==
function [Axel,Rvel] = Gimbal(Rate,Tin,Tst,Jg)    
% Gimbal Friction Dynamics
% Tin:  Input Torque (ft-lb)
% Rate: Gimbal Rate (rad/sec)
% Tfr:  Gimbal Friction Torque (ft-lb)
% axel: Gimbal Acceleration (ft/sec2)
% Tst:  Gimbal Static Friction Torq (ft-lb)
% Jg:   Gimbal Inertia (slg-ft^2)

if abs(Rate)<0.01                     % If Not Moving Much
    if abs(Tin)>Tst*1.05              % Exceeds Stiction, Start Moving
        Tfr=Tst*sign(Tin);            % Friction Torque resist motion
        Axel=(Tin-Tfr)/Jg;            % Gimbal Acceleration
        Rvel=0;
    else                              % Stop the Motion
        Axel=0;
        Tfr=0;                        % No Frict when not moving
        Rvel=1;                       % Reset Velocity to Zero
    end
    
else                                  % Gimbal is Fast Enough
    Tfr=Tst*sign(Rate);               % Friction Torque resist motion
    Axel=(Tin-Tfr)/Jg;                % Gimbal Acceleration
    Rvel=0;
end
